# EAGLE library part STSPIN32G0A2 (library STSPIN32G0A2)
Advanced brushless motor controller with embedded STM32G0 MCU Operating voltage from 6.7 to 45 V temperature range: -40 to +125 C Source: Datasheet
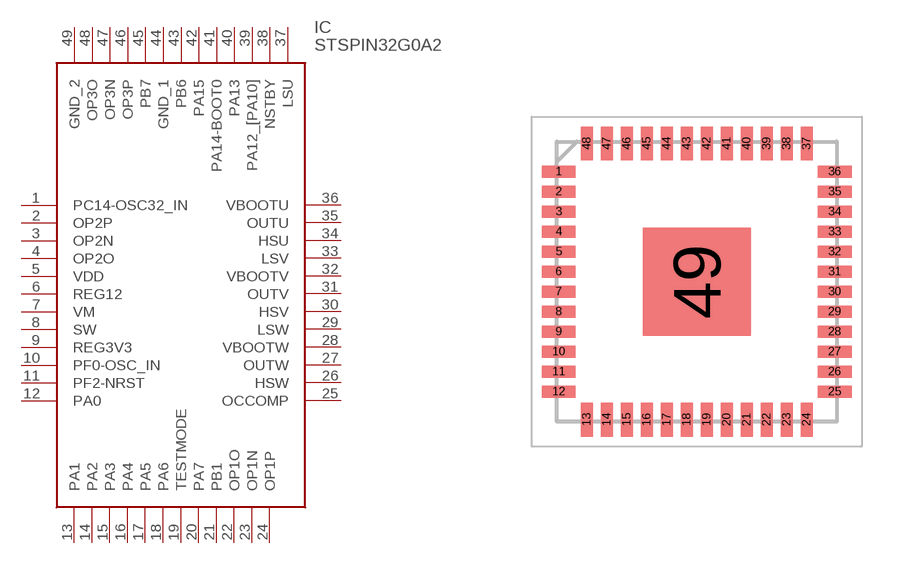
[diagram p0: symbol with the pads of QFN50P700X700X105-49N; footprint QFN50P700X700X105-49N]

Designator prefix IC

## STSPIN32G0A2 (Description: Advanced brushless motor controller with embedded STM32G0 MCU Operating voltage from 6.7 to 45 V temperature range: -40 to +125 C; Height: 1.05mm; Manufacturer_Name: STMicroelectronics; Manufacturer_Part_Number: STSPIN32G0A2)  [QFN50P700X700X105-49N]
1  PC14-OSC32_IN
2  OP2P
3  OP2N
4  OP2O
5  VDD
6  REG12
7  VM
8  SW
9  REG3V3
10  PF0-OSC_IN
11  PF2-NRST
12  PA0
13  PA1
14  PA2
15  PA3
16  PA4
17  PA5
18  PA6
19  TESTMODE
20  PA7
21  PB1
22  OP1O
23  OP1N
24  OP1P
25  OCCOMP
26  HSW
27  OUTW
28  VBOOTW
29  LSW
30  HSV
31  OUTV
32  VBOOTV
33  LSV
34  HSU
35  OUTU
36  VBOOTU
37  LSU
38  NSTBY
39  PA12_[PA10]
40  PA13
41  PA14-BOOT0
42  PA15
43  PB6
44  GND_1
45  PB7
46  OP3P
47  OP3N
48  OP3O
49  GND_2

## Footprint QFN50P700X700X105-49N (pad centres in mm)
VFQFPN 48 7x7x1.0 mm_2024
smd 0.85 x 0.3: 1 -3.45,2.75; 2 -3.45,2.25; 3 -3.45,1.75; 4 -3.45,1.25; 5 -3.45,0.75; 6 -3.45,0.25; 7 -3.45,-0.25; 8 -3.45,-0.75; 9 -3.45,-1.25; 10 -3.45,-1.75; 11 -3.45,-2.25; 12 -3.45,-2.75; 25 3.45,-2.75; 26 3.45,-2.25; 27 3.45,-1.75; 28 3.45,-1.25; 29 3.45,-0.75; 30 3.45,-0.25; 31 3.45,0.25; 32 3.45,0.75; 33 3.45,1.25; 34 3.45,1.75; 35 3.45,2.25; 36 3.45,2.75
smd 0.3 x 0.85: 13 -2.75,-3.45; 14 -2.25,-3.45; 15 -1.75,-3.45; 16 -1.25,-3.45; 17 -0.75,-3.45; 18 -0.25,-3.45; 19 0.25,-3.45; 20 0.75,-3.45; 21 1.25,-3.45; 22 1.75,-3.45; 23 2.25,-3.45; 24 2.75,-3.45; 37 2.75,3.45; 38 2.25,3.45; 39 1.75,3.45; 40 1.25,3.45; 41 0.75,3.45; 42 0.25,3.45; 43 -0.25,3.45; 44 -0.75,3.45; 45 -1.25,3.45; 46 -1.75,3.45; 47 -2.25,3.45; 48 -2.75,3.45
smd 2.7 x 2.7: 49 0,0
